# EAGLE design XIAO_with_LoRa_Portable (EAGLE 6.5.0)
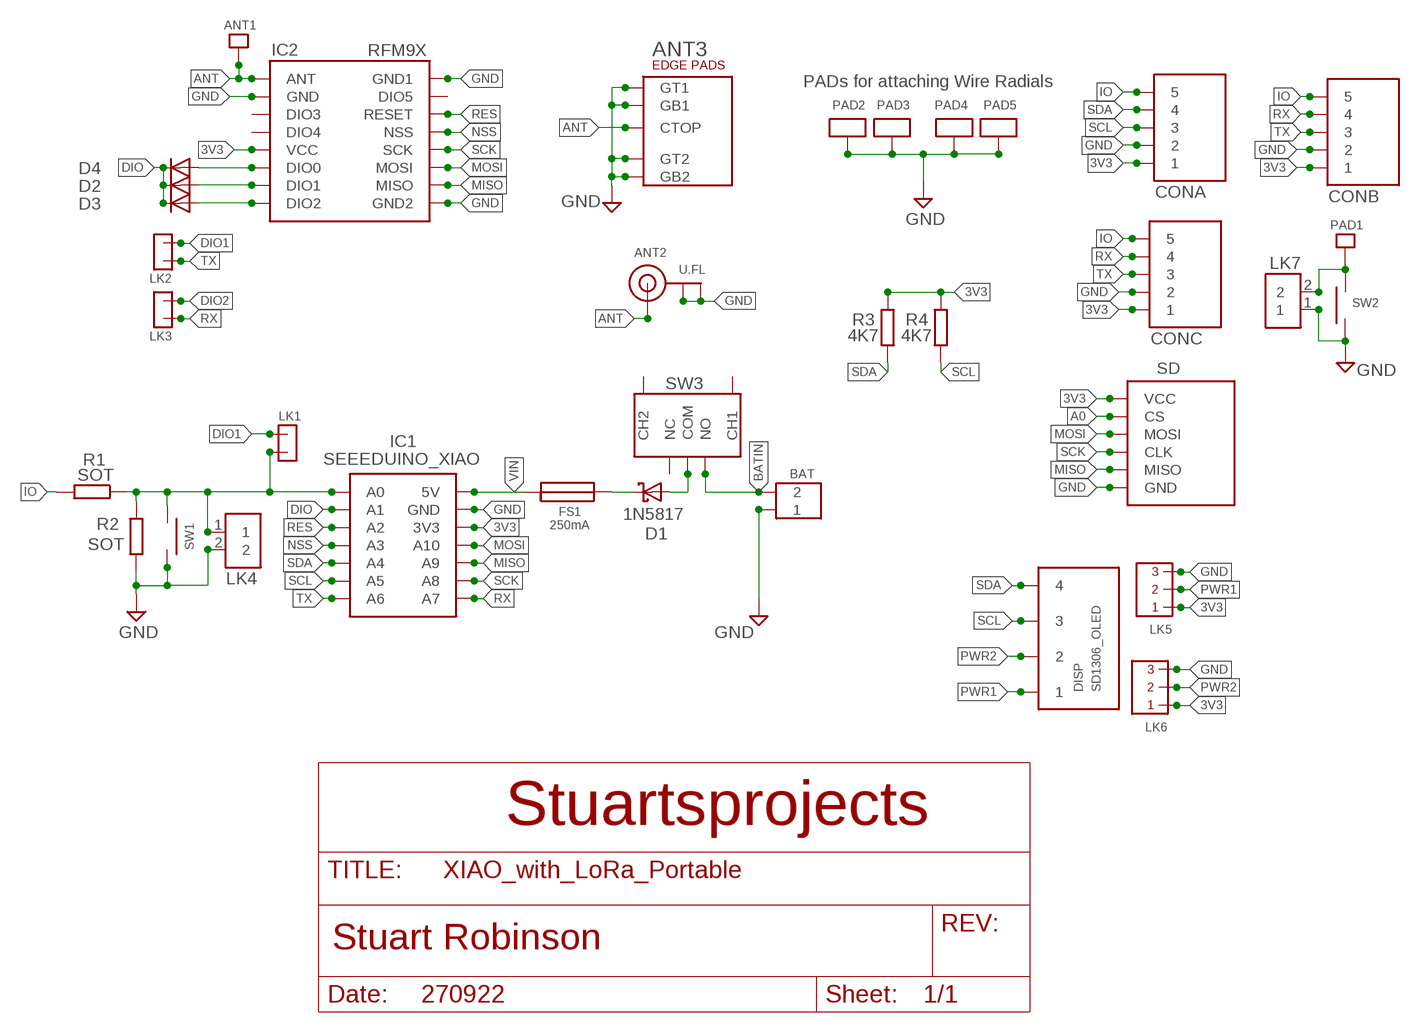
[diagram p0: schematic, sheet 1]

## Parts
ANT1  SINGLEPAD  [SINGLEPAD]
ANT2  U.FL  ANTENNA_U.FL2_DEFAULT  [U.FL2]
ANT3  SMA_EDGE  [SMA_EDGE]
BAT  SCREWTERMINAL_2WAY_0_1_INCH  [SCREWTERMINAL_2WAY_0_1_INCH]
CONA  5X1  [5X1]
CONB  5X1  [5X1]
CONC  5X1  [5X1]
D1  1N5817  1N5817-B  [DO41-7.6@1]
D2  1N4148  SIGNAL_DIODE_MIN  [SIGNAL_DIODE_MIN]
D3  1N4148  SIGNAL_DIODE_MIN  [SIGNAL_DIODE_MIN]
D4  1N4148  SIGNAL_DIODE_MIN  [SIGNAL_DIODE_MIN]
DISP  SD1306_OLED  [SD1306_OLED]
FS1  250mA  SMALL_POLYFUSE  [SMALL_POLYFUSE]
IC1  SEEEDUINO_XIAO  SEEEDUINO_XIAO_PIH  [SEEEDUINO_XIAO]
IC2  RFM9X  RFM98_PIH  [RFM98_PIH]
LK1  2PINMICROHEADER  [2PINMICROHEADER]
LK2  2PINMICROHEADER  [2PINMICROHEADER]
LK3  2PINMICROHEADER  [2PINMICROHEADER]
LK4  2X1  [2X1]
LK5  3PINMICROHEADER  [3PINMICROHEADER]
LK6  3PINMICROHEADER  [3PINMICROHEADER]
LK7  2X1  [2X1]
PAD1  SINGLEPAD  [SINGLEPAD]
PAD2  ANTPAD2  [ANTPAD2]
PAD3  ANTPAD2  [ANTPAD2]
PAD4  ANTPAD2  [ANTPAD2]
PAD5  ANTPAD2  [ANTPAD2]
R1  SOT  125MWRESISTOR  [125MWRESISTOR_MIN]
R2  SOT  125MWRESISTOR  [125MWRESISTOR_MIN]
R3  4K7  125MWRESISTOR  [125MWRESISTOR_MIN]
R4  4K7  125MWRESISTOR  [125MWRESISTOR_MIN]
SD  MICROSD_BREAKOUT2_DEFAULT  [MICROSD_BREAKOUT2]
SW1  SMTSWITCH_4_X_3_LARGE  [SMTSWITCH_4_X_3_LARGE]
SW2  SMTSWITCH_4_X_3_LARGE  [SMTSWITCH_4_X_3_LARGE]
SW3  SMALL_EDGE_SLIDE  [SMALL_EDGE_SLIDE]

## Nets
3V3 [POWER]: CONA.1 CONB.1 CONC.1 IC1.3V3 IC2.VCC LK5.1 LK6.1 R3.P$1 R4.P$1 SD.VCC
A0: IC1.D0(A0) LK1.2 LK4.1 R1.P$1 R2.P$1 SD.CS SW1.1
ANT: ANT1.P$1 ANT2.3(SIGNAL) ANT3.CTOP IC2.ANT
BATIN [POWER]: BAT.P$2 SW3.NO
DIO: D2.C D3.C D4.C IC1.D1(A1)
DIO0: D4.A IC2.DIO0
DIO1: D2.A IC2.DIO1 LK1.1 LK2.2
DIO2: D3.A IC2.DIO2 LK3.2
GND [POWER]: ANT2.1(GND) ANT2.2(GND) ANT3.GB1 ANT3.GB2 ANT3.GT1 ANT3.GT2 BAT.P$1 CONA.2 CONB.2 CONC.2 IC1.GND IC2.GND IC2.GND1 IC2.GND2 LK4.2 LK5.3 LK6.3 LK7.1 PAD2.P$1 PAD3.P$1 PAD4.P$1 PAD5.P$1 R2.P$2 SD.GND SW1.2 SW2.1
IO: CONA.5 CONB.5 CONC.5 R1.P$2
MISO: IC1.D9(A9) IC2.MISO SD.MISO
MOSI: IC1.D10(A10) IC2.MOSI SD.MOSI
N$1 [POWER]: LK7.2 PAD1.P$1 SW2.2
N$2 [POWER]: D1.A SW3.COM
NSS: IC1.D3(A3) IC2.NSS
POWERIN [POWER]: D1.C FS1.P$2
PWR1 [dispPower]: DISP.P$1 LK5.2
PWR2 [dispPower]: DISP.P$2 LK6.2
RES: IC1.D2(A2) IC2.RESET
RX: CONB.4 CONC.4 IC1.D7(A7) LK3.1
SCK: IC1.D8(A8) IC2.SCK SD.SCK(CLK)
SCL: CONA.3 DISP.P$3 IC1.D5(A5) R4.P$2
SDA: CONA.4 DISP.P$4 IC1.D4(A4) R3.P$2
TX: CONB.3 CONC.3 IC1.D6(A6) LK2.1
VIN [POWER]: FS1.P$1 IC1.5V
Unconnected: IC2.DIO3 IC2.DIO4 IC2.DIO5 SW3.CH1 SW3.CH2 SW3.NC

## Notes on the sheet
- PADs for attaching Wire Radials
- Stuartsprojects
- 270922

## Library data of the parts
ANT1 PAD1 = LMA2:SINGLEPAD
ANT2 = adafruit:ANTENNA_U.FL2
ANT3 = con-coax:SMA_EDGE
BAT = LMA2:SCREWTERMINAL_2WAY_0_1_INCH
CONA CONB CONC = My_Pin_Headers:5X1
D1 = diode:1N581*: 1.0A SCHOTTKY BARRIER RECTIFIER
D2-D4 = LMA2:SIGNAL_DIODE_MIN
DISP = LMA2:SD1306_OLED
FS1 = LMA2:SMALL_POLYFUSE
IC1 = LMA2:SEEEDUINO_XIAO
IC2 = LMA2:RFM98_PIH
LK1-LK3 = LMA2:2PINMICROHEADER
LK4 LK7 = My_Pin_Headers:2X1
LK5 LK6 = LMA2:3PINMICROHEADER
PAD2-PAD5 = LMA2:ANTPAD2
R1-R4 = LMA2:125MWRESISTOR
SD = LMA2:MICROSD_BREAKOUT2
SW1 SW2 = LMA2:SMTSWITCH_4_X_3
SW3 = switch-tact:SMALL_EDGE_SLIDE

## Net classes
0 default: width 0.254 mm
1 POWER: width 0.635 mm
2 VDD: width 0.635 mm
3 gpspower: width 0.635 mm
4 dispPower: width 0.635 mm

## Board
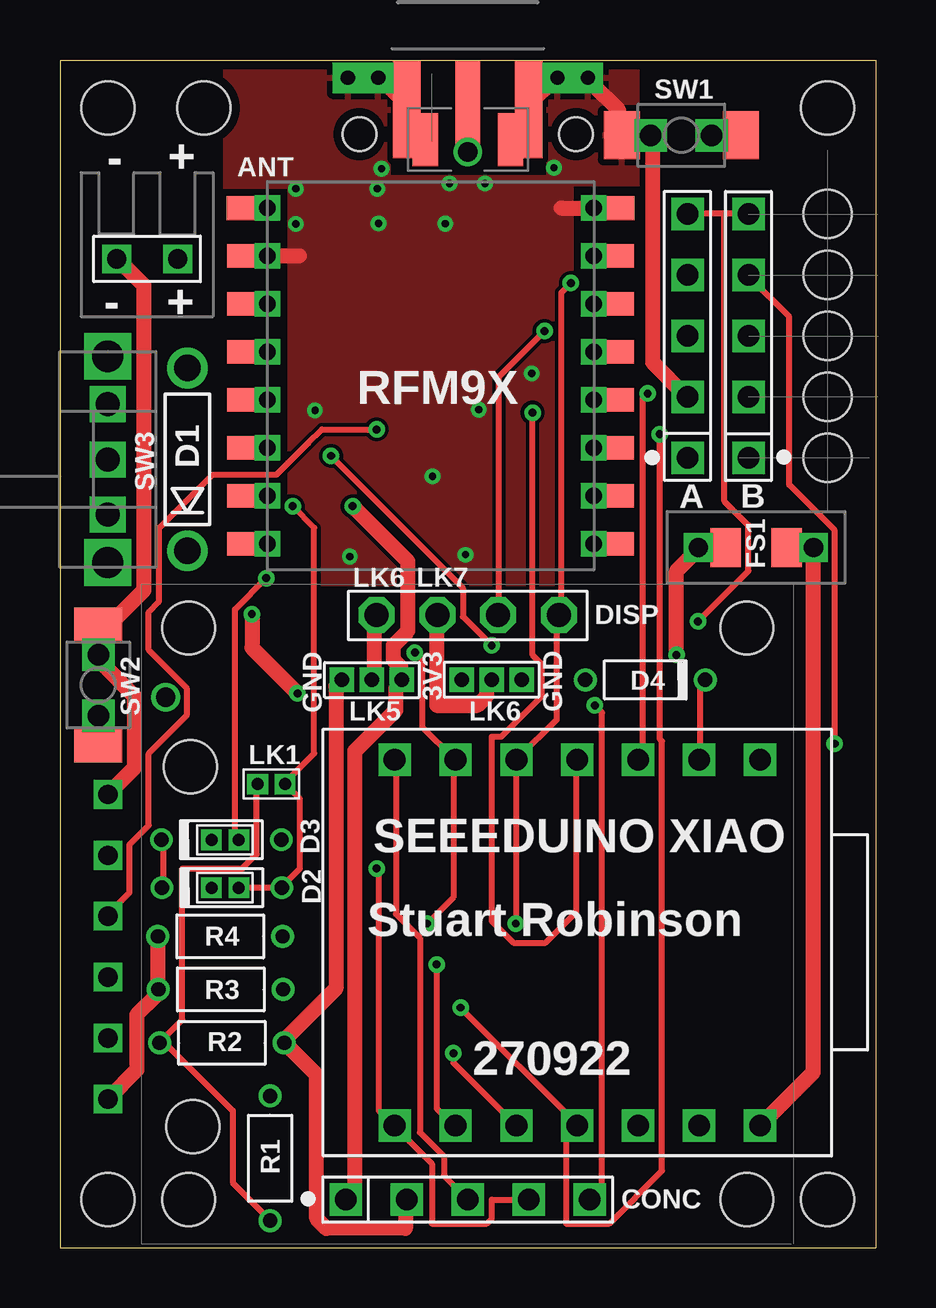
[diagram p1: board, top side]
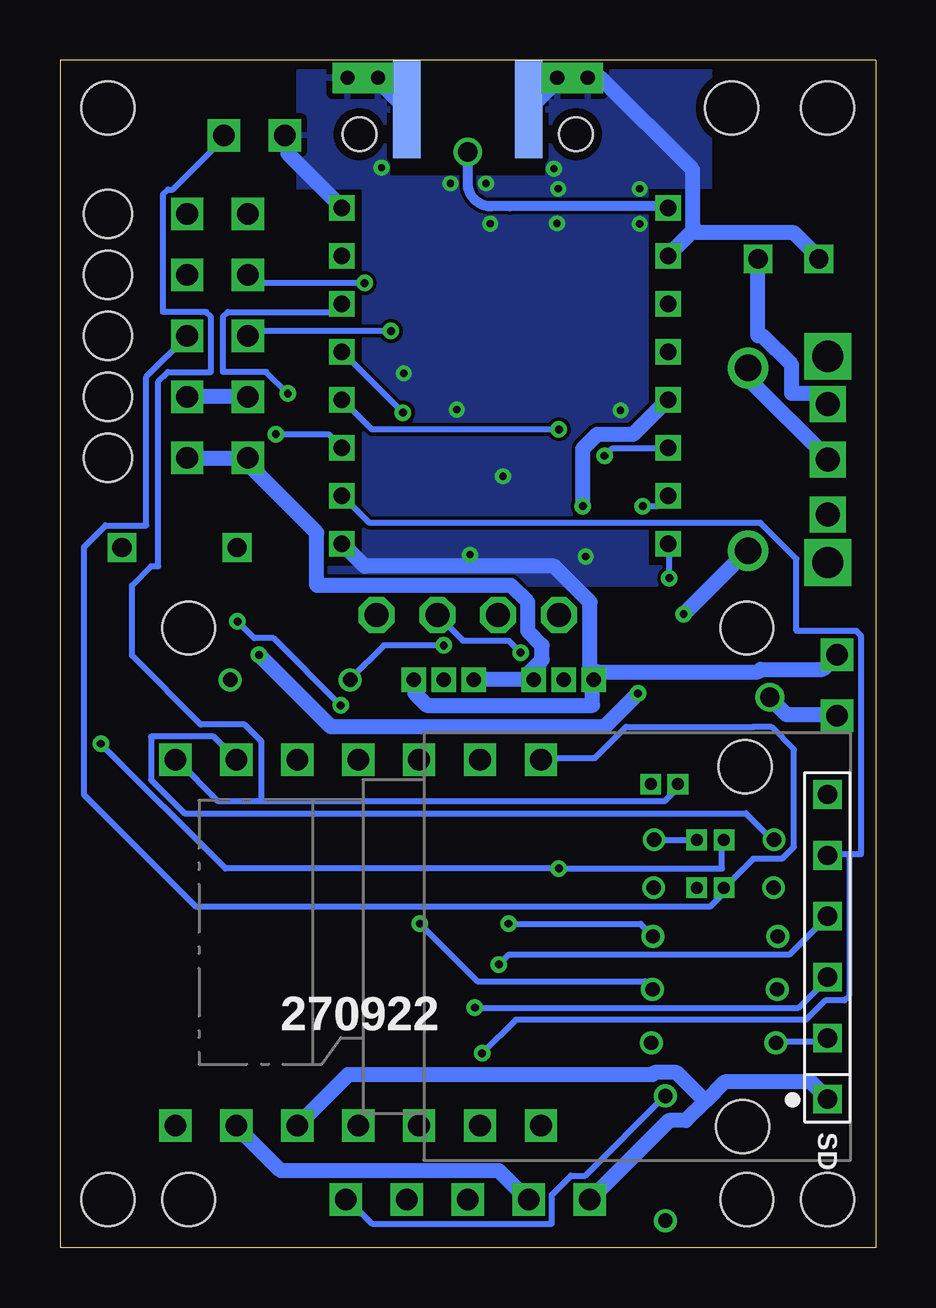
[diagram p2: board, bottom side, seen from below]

Size 34 x 49.5 mm. Coordinates in mm from the lower left corner, seen from the top.
Outline: 0,49.5 34,49.5 34,0 0,0 0,49.5
Copper layers (1*16): Top 0.0356mm / dielectric 1.5011mm / Bottom 0.0356mm
Design rules "LaenPCBOrder *": minimum track width 6mil, minimum drill 13mil, track to track 6mil, track to pad 6mil, pad to pad 6mil, via to via 6mil, smd to smd 6mil, copper to edge 15mil, drill to drill 6mil, minimum pad ring 7mil, minimum via ring 7mil, stop-mask expansion 4mil, vias tented up to drill 15mil, thermal gap 10mil
Holes 2.2 mm at 32,47.5 2,47.5 6,47.5 2,2 32,2
Holes 2 mm at 32,43.08 32,40.54 32,38 32,35.46 32,32.92
Holes 1.4 mm at 12.48,46.4 21.52,46.4
tRestrict: area 13.8,44.7 to 20.3,49.5; area 6.7,28.5 to 9.5,44.1; area 21.4,28.6 to 24.2,44.2
bRestrict: area 13.8,44.7 to 20.2,49.5; area 6.7,28.4 to 9.4,44.1; area 21.4,28.4 to 24.2,44.1

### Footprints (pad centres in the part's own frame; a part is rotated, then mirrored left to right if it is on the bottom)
SINGLEPAD = drill 0.8: P$1 0,0
U.FL2 = smd 2.2 x 1.05: 1 0,1.775; 2 0,-1.775 | smd 0.8 x 1: 3 1.525,0
SMA_EDGE = smd 4.064 x 1.016: CTOP -1.27,0 | smd 4.064 x 1.143 bottom: GB1 -1.27,2.54; GB2 -1.27,-2.54 | smd 4.064 x 1.143: GT1 -1.27,2.54; GT2 -1.27,-2.54
SCREWTERMINAL_2WAY_0_1_INCH = drill 0.8 square: P$1 -1.27,0; P$2 1.27,0
5X1 = drill 0.9 square: 1 -5.08,0; 2 -2.54,0; 3 0,0; 4 2.54,0; 5 5.08,0
DO41-7.6@1 = drill 1.1 pad 1.7: A 3.81,0; C -3.81,0
SIGNAL_DIODE_MIN = drill 0.6: A -2.5,0; C 2.5,0
SD1306_OLED = drill 1 pad 1.422 octagon: P$1 -3.81,12.455; P$2 -1.27,12.455; P$3 1.27,12.455; P$4 3.81,12.455 | hole 2.2: -11.63,11.91; 11.63,11.91; -11.63,-11.91; 11.63,-11.91
SMALL_POLYFUSE = drill 0.8 square: P$1 -2.4,0; P$2 2.4,0 | smd 1.27 x 1.635: P$3 -1.27,0; P$4 1.27,0
SEEEDUINO_XIAO = drill 0.9 square: 3V3 7.62,2.54; 5V 7.62,7.62; D0 -7.62,7.62; D1 -7.62,5.08; D2 -7.62,2.54; D3 -7.62,0; D4 -7.62,-2.54; D5 -7.62,-5.08; D6 -7.62,-7.62; D7 7.62,-7.62; D8 7.62,-5.08; D9 7.62,-2.54; D10 7.62,0; GND 7.62,5.08
RFM98_PIH = drill 0.7 pad 0.965 square: ANT -6.8,7.5; DIO0 -6.8,-2.5; DIO1 -6.8,-4.5; DIO2 -6.8,-6.5; DIO3 -6.8,3.5; DIO4 -6.8,1.5; DIO5 6.8,5.5; GND -6.8,5.5; GND2 6.8,-6.5; MISO 6.8,-4.5; MOSI 6.8,-2.5; NSS 6.8,1.5; RESET 6.8,3.5; SCK 6.8,-0.5; VCC -6.8,-0.5 | drill 0.7 pad 1.016 square: GND1 6.8,7.5 | smd 2.2 x 1: P$2 -7.4,7.5; P$6 7.4,7.5 | smd 2.159 x 0.965: P$4 -7.4,5.5; P$5 -7.4,1.5; P$7 7.4,5.5; P$9 -7.4,3.5; P$10 -7.4,-0.5; P$11 -7.4,-2.5; P$12 -7.4,-4.5; P$13 -7.4,-6.5; P$14 7.4,-6.5; P$15 7.4,-4.5; P$16 7.4,-2.5; P$17 7.4,-0.5; P$18 7.4,1.5; P$19 7.4,3.5
2PINMICROHEADER = drill 0.5 pad 0.8 square: 1 -0.06,0.575; 2 -0.06,-0.56
2X1 = drill 0.9 square: 1 -1.27,0; 2 1.27,0
3PINMICROHEADER = drill 0.6 pad 1.016 square: 1 0,-1.25; 2 0,0.001; 3 0,1.25
ANTPAD2 = drill 0.6 pad 1.27 square: P$1 0,0
125MWRESISTOR_MIN = drill 0.6: P$1 -2.6,0; P$2 2.6,0
MICROSD_BREAKOUT2 = drill 0.8 square: CS 3.81,0; GND -6.35,0; MISO -3.81,0; MOSI 1.27,0; SCK -1.27,0; VCC 6.35,0 | hole 2.2: -7.5,-3.44; 7.5,-3.54
SMTSWITCH_4_X_3_LARGE = smd 1.5 x 2: 1 -2.48,0; 2 2.48,0
SMALL_EDGE_SLIDE = drill 1.3 pad 1.85 square: CH1 -4.3,0; CH2 4.3,0 | drill 1 pad 1.422 square: COM 0,0; NC 2.3,0; NO -2.3,0

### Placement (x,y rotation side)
ANT1  17,45.67 0 top
ANT2  17,46.18 90 top
ANT3  17,48.7 90 top
BAT  3.63,41.21 0 top
CONA  26.16,38 90 top
CONB  28.7,38 90 top
CONC  17,2 0 top
D1  5.31,32.85 90 top
D2  6.75,15 180 top
D3  6.73,17 180 top
D4  24.4,23.66 0 top
DISP  17,13.91 0 top
FS1  29.02,29.18 180 top
IC1  21.57,12.71 270 top
IC2  15.45,35.83 0 top
LK1  8.8,19.26 270 top
LK2  6.89,15.06 90 top
LK3  6.89,17.05 90 top
LK4  25.9,46.36 180 top
LK5  13,23.66 90 top
LK6  18,23.66 270 top
LK7  1.6,23.44 270 top
PAD1  4.41,22.94 0 top
PAD2  12,48.76 0 top
PAD3  13.27,48.76 0 top
PAD4  20.74,48.76 0 top
PAD5  22.01,48.76 0 top
R1  8.76,3.72 90 top
R2  6.75,8.53 0 top
R3  6.7,10.76 0 top
R4  6.68,12.97 0 top
SD  2,12.54 270 bottom
SW1  25.9,46.36 180 top
SW2  1.6,23.45 270 top
SW3  1.99,32.85 270 top

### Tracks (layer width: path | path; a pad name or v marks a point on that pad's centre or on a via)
3V3  (via drill 0.33)
  Top 0.635: v12.2,30.9 14.5,28.6 14.5,25.7 13.9,25.1 13.9,24.5 14.2,24.2 14.2,23.7 LK5.1 14.1,23.4 14,23.3 14,22.4 12.3,20.7 12.3,2.3 12,2 CONC.1 | R4.P$1 4.1,12.9 4.1,10.8 R3.P$1 4,10.5 3.2,9.7 3.2,7.4 SD.VCC
  Bottom 0.635: CONB.1 28.7,32.9 26.2,32.9 CONA.1 26.1,32.6 23.3,29.8 23.3,27.6 15.2,27.6 14.5,26.9 14.5,25.7 13.9,25.1 13.9,24.5 14.4,24 LK5.1 14.3,23.7 16.7,23.7 LK6.1 | v12.2,30.9 12.2,33.3 11.6,33.9 10.1,33.9 8.7,35.3 IC2.VCC | 7.1,6.1 6.3,6.9 2.7,6.9 SD.VCC | 7.1,6.1 7.9,5.3 8.6,5.3 11.9,2 CONC.1 | IC1.3V3 22,7.2 9.3,7.2 9.2,7.3 8.3,7.3 7.3,6.3 7.1,6.1
A0
  Top 0.254: SW1.1 28.2,46.4 27.1,46.4 LK4.1 | LK1.2 8.2,19.3 8.2,16.4 7.6,15.8 5.1,15.8 5.1,9.5 4.2,8.6 R2.P$1 4.3,8.6 7.2,5.7 7.2,2.7 8.7,1.2 R1.P$1
  Bottom 0.254: SD.CS 2,8.7 2.1,8.6 4.1,8.6 R2.P$1 | 25.6,18.6 8.8,18.6 8.3,19.1 8.3,19.3 LK1.2 | 25.6,18.6 27.4,18.6 29.1,20.3 IC1.D0 | LK4.1 27.1,46.3 29.3,44.1 29.5,44.1 29.7,43.9 29.7,39 27.9,39 27.7,38.8 27.7,36.5 29.5,36.5 29.9,36.1 29.9,28.4 30.2,28.4 31,27.6 31,24.67 28.13,21.8 26.3,21.8 25.6,21.1 25.6,18.7 25.6,18.6
ANT
  Top 0.254: ANT3.CTOP 17,47.5 ANT2.3 17,47.4 17,45.7 ANT1.P$1
  Bottom 0.254: 8.7,43.4 IC2.ANT | 17,45.6 ANT1.P$1
  Bottom 0.406: 8.7,43.4 15.24,43.4 16.03,43.4 arc90 17,44.37 ANT1.P$1
BATIN
  Bottom 0.635: BAT.P$2 4.9,38 4.7,38 3.5,36.8 3.5,35.6 2.4,35.6 2,35.2 SW3.NO
DIO
  Top 0.254: D2.C 4.3,15 4.3,17 D3.C | D4.C 26.9,23.6 26.7,23.4 26.7,20.4 IC1.D1
  Bottom 0.254: D3.C 4.3,17 5.4,18.1 28.8,18.1 30.2,19.5 30.2,21.3 27.6,21.3 26.7,20.4 IC1.D1
DIO0  (via drill 0.33)
  Top 0.254: v18,25.1 16.8,26.3 16.8,27.5 v11.3,33
  Bottom 0.254: v18,25.1 20.5,25.1 21.9,23.7 D4.A | v11.3,33 11,33.3 8.7,33.3 IC2.DIO0
DIO1  (via drill 0.33)
  Top 0.254: LK2.2 7.5,15 9.2,15 D2.A 9.3,15.1 10,15.8 10,18.7 9.4,19.3 LK1.1 9.4,19.4 10.6,20.6 10.6,30 v9.7,30.9
  Bottom 0.254: v9.7,30.9 9.1,30.9 8.7,31.3 IC2.DIO1
DIO2  (via drill 0.33)
  Top 0.254: v8.6,27.9 7.3,26.6 7.3,17.1 7.4,17 LK3.2
  Bottom 0.254: LK3.2 7.5,17 9.2,17 D3.A | v8.6,27.9 8.6,29.3 IC2.DIO2
GND  (via drill 0.3)
  Top 0.635: PAD2.P$1 12,48.8 13.2,48.8 PAD3.P$1 13.5,48.6 14.3,47.8 14.3,47.7 ANT3.GB1 14.5,47.4 14.5,46.9 15.2,46.2 ANT2.1 | ANT2.2 18.8,46.2 19.5,46.9 19.5,47.4 ANT3.GT2 19.7,47.7 19.7,47.8 20.5,48.6 PAD4.P$1 20.8,48.8 22,48.8 PAD5.P$1 22.2,48.5 23.3,47.4 23.3,46.7 SW1.2 23.4,46.4 24.5,46.4 LK4.2 24.7,46.1 24.7,36.9 26.1,35.5 CONA.2 | CONC.2 14.4,2 14.4,0.8 11.1,0.8 10.7,1.2 10.7,7.2 9.4,8.5 R2.P$2 9.5,8.8 11.5,10.8 11.5,23.4 11.7,23.6 LK5.3 | SD.GND 3.1,20 3.1,23 1.7,24.4 LK7.1 1.6,24.8 1.6,25.9 SW2.1 1.9,25.8 3.5,27.4 3.5,40.1 2.4,41.2 BAT.P$1 | IC2.GND 9.97,41.34 | 20.9,43.33 22.22,43.33
  Bottom 0.635: 7.7,42.3 8.6,41.4 IC2.GND | 7.7,42.3 3.4,42.3 2.4,41.3 BAT.P$1 | PAD3.P$1 13.2,48.7 14.4,47.5 ANT3.GB1 14.7,47.6 | 7.7,42.3 7.6,42.6 7.62,42.6 7.62,44.78 7.62,44.92 11.47,48.77 PAD2.P$1 12,48.7 | PAD4.P$1 20.8,48.7 19.6,47.5 ANT3.GT2 19.3,47.6 | CONA.2 26.2,35.5 28.7,35.5 CONB.2 | IC2.GND1 22.3,43.4 24.5,45.6 24.5,46.3 LK4.2 | IC1.GND 26.6,5 24.8,3.2 15.7,3.2 14.5,2 CONC.2 | LK5.3 11.8,23.6 11.8,22.6 18.7,22.6 19.2,23.1 19.2,23.6 LK6.3 | IC2.GND2 22.2,29.3 21.3,28.4 13.4,28.4 11.9,26.9 11.9,23.9 LK5.3 | LK7.1 2.2,24.1 4.8,24.1 4.9,24 11.6,24 LK5.3
  other vias: 16.24,44.35 17.72,44.35 9.83,44.13 9.83,42.67 13.23,44.13 13.28,42.69 16.06,42.68 20.59,45.01 13.41,44.97 19.67,36.44 15.53,32.15 12.08,28.8 16.91,28.88 17.46,34.93 10.63,34.9
  pour Bottom: 6.9,49.5 24.06,49.5 24.06,27.66 6.9,27.66
  pour Top: 6.9,49.5 24.06,49.5 24.06,27.66 6.9,27.66
IO  (via drill 0.33)
  Top 0.254: 27.7,43.1 28.7,43.1 CONB.5 | 27.7,43.1 26.2,43.1 CONA.5 | v26.6,26.1 28.7,28.2 28.7,30.1 27.7,31.1 27.7,43 27.7,43.1 | v22.3,22.6 22.6,22.3 22.6,2.5 22.1,2 CONC.5
  Bottom 0.254: R1.P$2 8.8,6.3 12.1,3 12.7,3 13.5,2.2 13.5,1 21,1 22,2 CONC.5 | v26.6,26.1 25.9,25.4 25.1,25.4 v22.3,22.6
MISO  (via drill 0.33)
  Top 0.254: v16.4,8.1 16.4,7.7 19,5.1 IC1.D9
  Bottom 0.254: 1.1,16.4 2,16.4 SD.MISO | 1.1,16.4 0.6,16.4 0.6,25.5 0.8,25.7 3.3,25.7 3.3,28.7 4.8,30.2 21.1,30.2 22.2,31.3 IC2.MISO | v16.4,8.1 15,9.5 2.9,9.5 2.1,10.3 1.3,10.3 1.1,10.5 1.1,16.3 1.1,16.4
MOSI  (via drill 0.33)
  Top 0.254: v25,33.9 25,21.2 25.1,21.1 25.1,3.2 22.9,1 21.1,1 21.1,4.6 21.5,5 IC1.D10 21.5,5.2 v16.7,10
  Bottom 0.254: v25,33.9 22.8,33.9 22.3,33.4 IC2.MOSI | v16.7,10 3.2,10 2,11.2 SD.MOSI
N$1
  Top 0.635: SW2.2 1.6,21 1.6,22.1 LK7.2
  Bottom 0.635: PAD1.P$1 4.4,22.9 3.7,22.2 1.6,22.2 LK7.2
N$2
  Bottom 0.635: SW3.COM 2,32.9 5.3,36.2 5.3,36.6 D1.A
NSS  (via drill 0.33)
  Top 0.254: v19.7,34.8 19.7,24.7 20.1,24.3 20.1,23 18.4,21.3 18,21.3 18,13.6 18.9,12.7 20.24,12.7 21.5,13.96 21.5,20.3 IC1.D3
  Bottom 0.254: v19.7,34.8 22.2,37.3 IC2.NSS
POWERIN  (via drill 0.33)
  Top 0.635: v25.7,24.7 25.7,28.2 26.6,29.1 FS1.P$2 | v9.9,23.1 8,25 v8,26.4
  Bottom 0.635: v25.7,24.7 22.7,21.7 11.3,21.7 v9.9,23.1 | v8,26.4 5.4,29 D1.C
PWR1
  Top 0.635: LK5.2 13,23.7 13.1,23.8 13.1,26.3 DISP.P$1
PWR2
  Top 0.635: LK6.2 18,23.6 17.8,23.4 17.8,23 17.4,22.6 15.7,22.6 15.7,26.3 DISP.P$2
RES  (via drill 0.33)
  Top 0.254: v24.5,35.6 24.3,35.4 24.3,20.5 24.2,20.4 IC1.D2
  Bottom 0.254: v24.5,35.6 25.4,36.5 27.2,36.5 27.2,38.8 27,39 22.6,39 22.3,39.3 IC2.RESET
RX  (via drill 0.33)
  Top 0.254: v13.2,15.8 13.3,15.7 13.3,5.7 13.9,5.1 IC1.D7 14,5 15.5,3.5 15.5,1 17.8,1 18,1.2 18,2 19.5,2 CONC.4 | v32.3,21 32.3,29.9 30.4,31.8 30.4,38.8 28.7,40.5 CONB.4
  Bottom 0.254: LK3.1 6.4,16.9 6.4,15.8 v13.2,15.8 13.3,15.8 27.1,15.8 v32.3,21
SCK  (via drill 0.33)
  Top 0.254: SD.SCK 2,13.9 2.9,14.8 2.9,16.8 3.7,17.6 3.7,20.6 5.3,22.2 5.3,23.3 3.7,24.9 3.7,26.5 4.1,26.9 4.11,26.91 4.11,29.96 6.35,32.2 9,32.2 9.5,32.7 9.52,32.7 10.35,33.53 10.92,34.1 v13.2,34.1 | v15.7,11.8 15.7,5.8 16.4,5.1 IC1.D8
  Bottom 0.254: v13.2,34.1 21,34.1 22.2,35.3 IC2.SCK | v15.7,11.8 15.3,12.2 3.6,12.2 SD.SCK
SCL  (via drill 0.33)
  Top 0.254: v15.3,13.5 16.4,14.6 16.4,20.3 IC1.D5 16.4,20.4 15.1,21.7 15.1,24.5 v14.8,24.8 | v20.2,38.2 18.3,36.3 18.3,26.4 DISP.P$3
  Bottom 0.254: v15.3,13.5 9.8,13.5 9.3,13 R4.P$2 | v20.2,38.2 25.9,38.2 26.1,38 CONA.3 | v14.8,24.8 15.3,25.3 17.2,25.3 18.2,26.3 DISP.P$3
SDA  (via drill 0.33)
  Top 0.254: v19,13.5 19,20.3 IC1.D4 19.1,20.4 20.7,22 20.7,26.3 DISP.P$4 20.9,26.4 20.9,39.8 v21.3,40.2
  Bottom 0.254: v19,13.5 16.6,11.1 9.6,11.1 9.3,10.8 R3.P$2 | v21.3,40.2 25.8,40.2 26.1,40.5 CONA.4
TX
  Top 0.254: CONC.3 16,3 16,3.8 15,4.8 15,12.9 14,13.9 14,20.3 IC1.D6
  Bottom 0.254: IC1.D6 13.9,20.4 11.7,20.4 10.4,21.7 5.1,21.7 5.09,21.69 4.33,21.69 3.4,20.76 3.4,16.7 3.9,16.2 5.1,16.2 LK2.1 6.3,14.9 6.3,14.8 6.9,14.2 28.33,14.2 33,18.87 33,29.2 32.1,30.1 30.4,30.1 30.4,36.3 CONB.3
VIN
  Top 0.635: FS1.P$1 31.4,29.1 31.4,7.3 IC1.5V

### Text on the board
tNames: SW1 | - | + | ANT | - | + | RFM9X | SW3 | D1 | A | B | FS1 | LK6 | LK7 | DISP | SW2 | GND | 3V3 | GND | D4 | LK5 | LK6 | LK1 | D3 | SEEEDUINO XIAO | D2 | R4 | Stuart Robinson | R3 | R2 | 270922 | R1 | CONC
bNames: 270922 | SD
